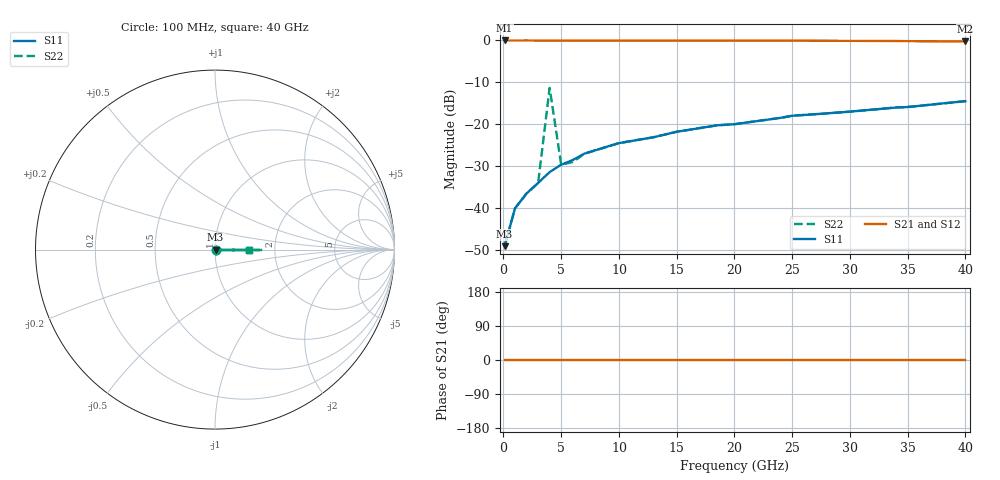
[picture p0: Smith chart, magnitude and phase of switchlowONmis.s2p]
# GHZ S MA R 50
!Output file by Shape3_28
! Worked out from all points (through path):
!   20 points, 100 MHz to 40 GHz, reference 50 ohm
!   highest |S21| = -0.09 dB at 100 MHz (marker M1); lowest = -0.3 dB at 40 GHz (marker M2)
!   lowest |S11| = -49.0 dB at 100 MHz (marker M3), VSWR 1.01, Z = 50.4 + j0 ohm
!   |S11| at or under -10 dB: start of sweep to end of sweep
!   |S22| runs from -49.0 to -11.4 dB; largest |S21 - S12| = 0.018
0.1  0.003548 0.0  0.99 0.0  0.99 0.0  0.003548 0.0
1  0.01 0.0  0.988 0.0  0.988 0.0  0.01 0.0
2  0.015 0.0  0.99 0.0  0.99 0.0  0.015 0.0
3  0.02 0.0  0.987 0.0  0.987 0.0  0.02 0.0
4  0.027 0.0  0.986 0.0  0.986 0.0  0.27 0.0
5  0.033 0.0  0.986 0.0  0.986 0.0  0.033 0.0
6  0.0375 0.0  0.985 0.0  0.985 0.0  0.0355 0.0
7  0.0446 0.0  0.985 0.0  0.985 0.0  0.0446 0.0
10  0.0596 0.0  0.985 0.0  0.985 0.0  0.0596 0.0
13  0.07 0.0  0.986 0.0  0.986 0.0  0.07 0.0
15  0.0813 0.0  0.987 0.0  0.987 0.0  0.0813 0.0
18.5  0.097 0.0  0.986 0.0  0.986 0.0  0.097 0.0
20  0.1 0.0  0.985 0.0  0.985 0.0  0.1 0.0
24  0.119 0.0  0.984 0.0  0.984 0.0  0.119 0.0
25  0.126 0.0  0.984 0.0  0.984 0.0  0.126 0.0
27.5  0.133 0.0  0.981 0.0  0.981 0.0  0.133 0.0
30  0.141 0.0  0.979 0.0  0.979 0.0  0.141 0.0
34  0.158 0.0  0.975 0.0  0.957 0.0  0.158 0.0
35  0.16 0.0  0.971 0.0  0.971 0.0  0.16 0.0
40  0.188 0.0  0.965 0.0  0.965 0.0  0.188 0.0
